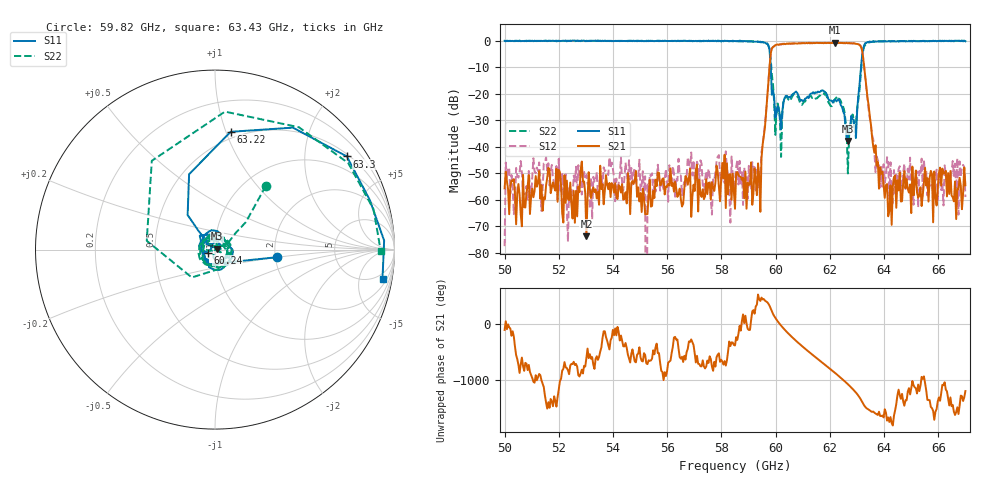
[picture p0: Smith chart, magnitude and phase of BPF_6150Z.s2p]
!Agilent Technologies,E8361A,US42410132,A.06.03.05
!Agilent E8361A: A.06.03.05
!Date: Friday, July 11, 2008 14:46:56
!Correction: S11(Full 2 Port(1,2)) S21(Full 2 Port(1,2)) S12(Full 2 Port(1,2)) S22(Full 2 Port(1,2))
!S2P File: Measurements: S11, S21, S12, S22:
# Hz S  MA  R 50
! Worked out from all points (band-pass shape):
!   401 points, 50 GHz to 67 GHz, reference 50 ohm
!   highest |S21| = -0.74 dB at 62.2 GHz (marker M1); lowest = -73.8 dB at 53.02 GHz (marker M2)
!   |S21| within 3 dB of the highest: 59.84 GHz to 63.19 GHz (3.347 GHz wide, 5.44 % of centre)
!   lowest |S11| = -37.8 dB at 62.66 GHz (marker M3), VSWR 1.03, Z = 51.2 + j0.564 ohm
!   |S11| at or under -10 dB: 59.82 GHz to 63.15 GHz (3.33 GHz wide, 5.42 % of centre)
!   |S22| runs from -50.1 to 0.1 dB; largest |S21 - S12| = 0.023
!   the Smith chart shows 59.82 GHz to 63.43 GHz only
!   S11 on the Smith chart (normalised r, x): 59.82 GHz: 2.03, -0.20; 60.24 GHz: 0.92, -0.03; 63.22 GHz: 0.44, +1.04; 63.3 GHz: 0.56, +3.06; 63.43 GHz: 3, -11
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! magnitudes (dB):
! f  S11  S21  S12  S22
! 50 GHz  0.0  -55.7  -77.5  0.0
! 50.13 GHz  -0.1  -55.9  -47.8  -0.2
! 51.53 GHz  0.1  -54.5  -43.9  -0.1
! 52.38 GHz  -0.1  -60.1  -55.3  -0.1
! 52.59 GHz  0.1  -68.7  -53.1  -0.2
! 52.85 GHz  0.0  -45.6  -58.0  0.0
! 53.02 GHz  -0.1  -73.8  -50.6  0.0
! 55.7 GHz  -0.2  -49.8  -52.1  0.0
! 58.5 GHz  -0.1  -63.4  -52.4  -0.2
! 59.35 GHz  -0.4  -46.3  -55.2  -0.3
! 59.82 GHz  -9.2  -4.9  -4.9  -6.9
! 60.24 GHz  -27.0  -1.3  -1.1  -28.2
! 61.35 GHz  -19.9  -1.0  -0.9  -21.6
! 62.2 GHz  -22.2  -0.7  -0.9  -22.0
! 62.66 GHz  -37.8  -1.0  -0.9  -50.1
! 62.96 GHz  -36.7  -1.2  -1.1  -30.9
! 63.22 GHz  -3.6  -5.6  -5.6  -4.3
! 63.3 GHz  -0.9  -13.2  -13.6  -1.7
! 63.43 GHz  -0.5  -24.3  -25.9  -0.7
! 63.77 GHz  -0.2  -45.7  -45.0  -0.3
! 64.19 GHz  -0.2  -64.1  -59.7  -0.1
! 67 GHz  -0.2  -54.5  -59.0  -0.2
